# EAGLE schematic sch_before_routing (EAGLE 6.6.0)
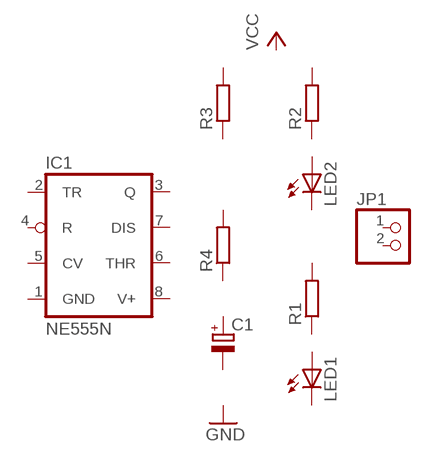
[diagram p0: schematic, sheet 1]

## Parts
C1  CPOL-EUE2.5-6  [E2,5-6]
IC1  NE555N  [DIL08]
JP1  PINHD-1X2  [1X02]
LED1  LED5MM  [LED5MM]
LED2  LED5MM  [LED5MM]
R1  R-EU_0207/10  [0207/10]
R2  R-EU_0207/10  [0207/10]
R3  R-EU_0207/10  [0207/10]
R4  R-EU_0207/10  [0207/10]
Unconnected: C1.+ C1.- IC1.2(TR) IC1.3(Q) IC1.4(R) IC1.5(CV) IC1.6(THR) IC1.7(DIS) JP1.1 JP1.2 LED1.A LED1.K(C) LED2.A LED2.K(C) R1.1 R1.2 R2.1 R2.2 R3.1 R3.2 R4.1 R4.2

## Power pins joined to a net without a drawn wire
GND: IC1.1(GND)
V+: IC1.8(V+)

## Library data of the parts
C1 = rcl:CPOL-EU: POLARIZED CAPACITOR, European symbol
IC1 = linear:*555: TIMER
JP1 = pinhead:PINHD-1X2: PIN HEADER
LED1 LED2 = led:LED: LED
R1-R4 = rcl:R-EU_: RESISTOR, European symbol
